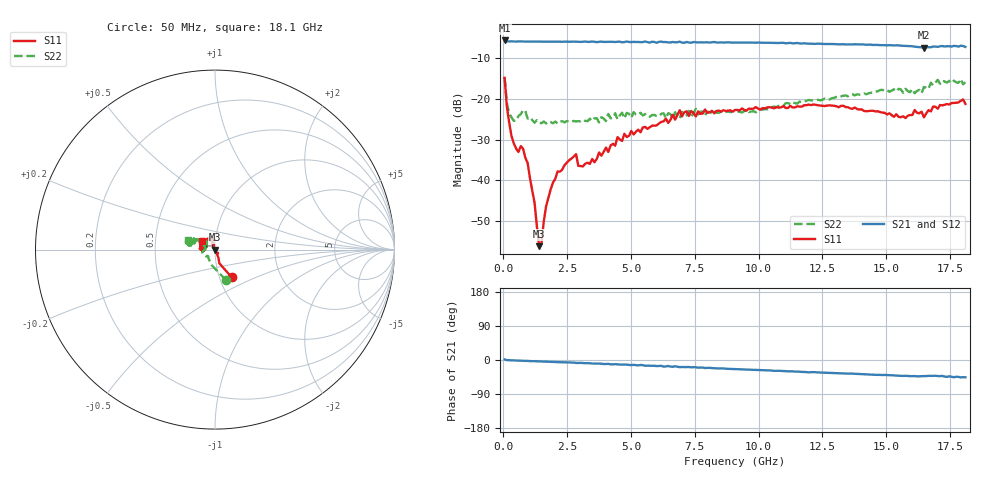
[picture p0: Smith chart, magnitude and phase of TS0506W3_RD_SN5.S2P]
! Network Analyzer HP8720D.06.14 Serial No. US36140669
! 30 Sep 2005  13:43:07
! Frequency  S11  S21  S12  S22
# HZ  S  DB R 50
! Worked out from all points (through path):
!   201 points, 50 MHz to 18.1 GHz, reference 50 ohm
!   highest |S21| = -5.68 dB at 50 MHz (marker M1); lowest = -7.4 dB at 16.48 GHz (marker M2)
!   group delay of S21, straight-line fit = 7.23 ps
!   lowest |S11| = -56.1 dB at 1.404 GHz (marker M3), VSWR 1.00, Z = 49.9 - j0.121 ohm
!   |S11| at or under -10 dB: start of sweep to end of sweep
!   |S22| runs from -26.0 to -14.8 dB; largest |S21 - S12| = 0.015
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5e7  -14.82 -58.9  -5.68 1.5  -5.70 1.8  -14.82 -70.2
1.4025e8  -21.96 -72.3  -5.91 -0.4  -5.86 -0.4  -21.10 -102.5
4.11e8  -30.92 -63.7  -5.93 -1.2  -5.92 -1.0  -25.40 -134.4
7.72e8  -32.18 -57.2  -5.96 -2.3  -5.93 -2.2  -22.76 -166.2
9.525e8  -35.72 -81.4  -5.95 -2.3  -5.95 -2.4  -24.84 -178.2
1.22325e9  -45.49 -92.0  -5.97 -3.1  -5.96 -3.2  -25.84 174.0
1.40375e9  -56.10 -129.3  -5.94 -3.7  -5.95 -3.5  -25.85 175.0
1.494e9  -55.36 148.3  -5.97 -3.9  -5.95 -4.0  -25.96 169.8
1.6745e9  -46.34 117.6  -5.95 -4.3  -5.95 -4.3  -26.02 169.6
2.12575e9  -37.77 110.4  -5.95 -5.7  -5.96 -5.5  -26.04 161.7
2.84775e9  -33.54 124.2  -5.99 -7.7  -5.98 -7.5  -25.52 149.3
3.1185e9  -36.56 133.2  -5.98 -8.0  -5.97 -8.2  -25.14 167.2
4.47225e9  -29.38 102.8  -5.99 -11.5  -6.00 -11.1  -25.03 160.8
6.09675e9  -26.02 108.1  -6.01 -15.6  -5.93 -15.5  -24.32 151.8
6.909e9  -22.78 111.7  -5.97 -18.9  -6.07 -18.2  -24.85 139.4
7.54075e9  -24.30 110.2  -6.12 -19.1  -5.97 -19.8  -22.45 145.3
9.075e9  -22.71 135.1  -6.18 -23.9  -6.13 -23.7  -23.05 138.8
1.21435e10  -21.38 176.5  -6.49 -31.9  -6.44 -31.9  -20.40 152.6
1.512175e10  -23.52 -176.5  -6.84 -40.1  -6.75 -39.4  -18.25 156.8
1.64755e10  -24.51 167.9  -7.42 -42.7  -7.32 -41.8  -17.07 161.1
1.68365e10  -21.86 164.6  -7.17 -41.8  -7.25 -42.0  -16.68 171.8
1.81e10  -21.24 148.6  -7.26 -45.6  -7.22 -46.9  -15.91 159.6
